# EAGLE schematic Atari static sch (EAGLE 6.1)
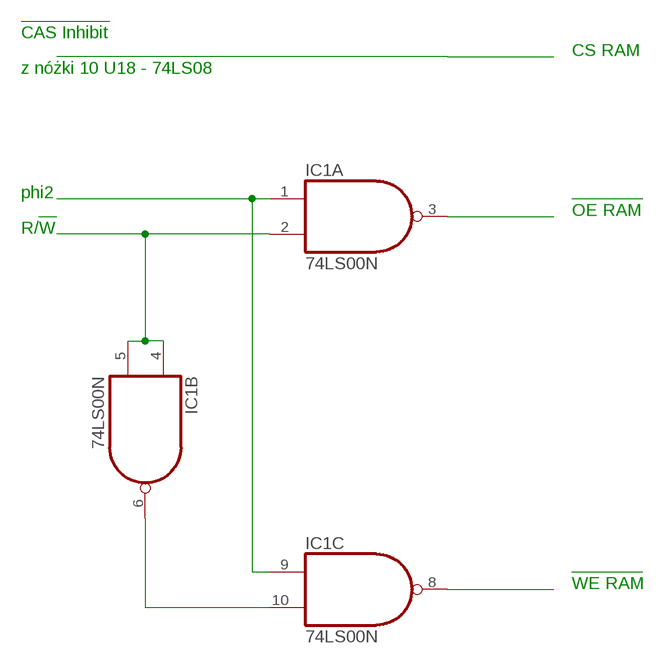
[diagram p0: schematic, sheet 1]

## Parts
IC1  74LS00N  [DIL14]

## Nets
N$1: IC1.1(A:I0) IC1.9(C:I0)
N$2: IC1.2(A:I1) IC1.4(B:I0) IC1.5(B:I1)
N$3: IC1.6(B:O) IC1.10(C:I1)
N$4: IC1.3(A:O)
N$5: IC1.8(C:O)
Unconnected: IC1.11(D:O) IC1.12(D:I0) IC1.13(D:I1)

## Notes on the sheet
- CAS Inhibit
- CS RAM
- z nóżki 10 U18 - 74LS08
- phi2
- OE RAM
- R/W
- WE RAM

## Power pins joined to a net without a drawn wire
GND: IC1.7(P:GND)
VCC: IC1.14(P:VCC)

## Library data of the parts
IC1 = 74xx-us:74*00: Quad 2-input NAND gate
